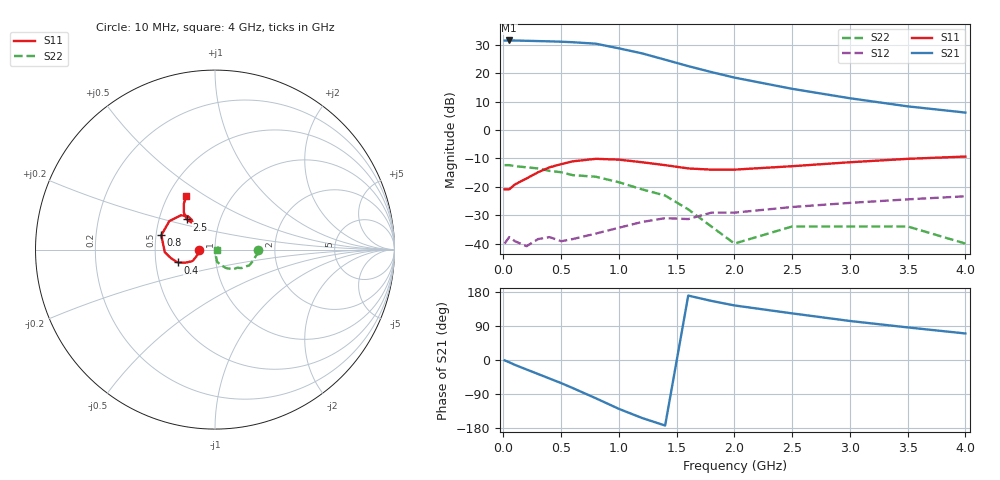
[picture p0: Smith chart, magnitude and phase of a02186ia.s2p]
!  INA-02186  S PARAMETERS
!  Id = 35 mA  LAST UPDATED 07-22-92
# ghz s ma r 50
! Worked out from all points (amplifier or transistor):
!   19 points, 10 MHz to 4 GHz, reference 50 ohm
!   highest |S21| = 31.5 dB at 50 MHz (marker M1)
!   |S21| within 3 dB of that: start of sweep to 1.025 GHz
!   unconditionally stable (mu >= 1): start of sweep to end of sweep
!   at 200 MHz: K = 1.59, MAG = 31.6 dB, |S12| = -40.9 dB
!   at 1 GHz: K = 1.16, MAG = 29.2 dB, |S12| = -34.4 dB
!   at 4 GHz: K = 3.28, MAG = 6.7 dB, |S12| = -23.3 dB
!   S11 on the Smith chart (normalised r, x): 10 MHz: 0.83, -0.01; 400 MHz: 0.65, -0.10; 800 MHz: 0.53, +0.09; 2.5 GHz: 0.69, +0.25; 4 GHz: 0.62, +0.42
0.01  0.09 -178.0  37.38 -1.0  0.01 1.0  0.24 -1.0
0.05  0.09 -172.0  37.55 -6.0  0.013 11.0  0.24 -5.0
0.1  0.11 -160.0  37.46 -13.0  0.011 8.0  0.23 -9.0
0.2  0.14 -153.0  37.04 -25.0  0.009 15.0  0.22 -17.0
0.3  0.18 -156.0  36.62 -37.0  0.012 1.0  0.21 -25.0
0.4  0.22 -161.0  36.2 -49.0  0.013 28.0  0.19 -30.0
0.5  0.25 -169.0  35.7 -61.0  0.011 42.0  0.18 -35.0
0.6  0.28 -177.0  34.94 -74.0  0.012 44.0  0.16 -39.0
0.8  0.31 165.0  32.93 -101.0  0.015 52.0  0.15 -47.0
1  0.3 148.0  27.26 -129.0  0.019 57.0  0.12 -59.0
1.2  0.27 135.0  22.26 -153.0  0.024 62.0  0.09 -70.0
1.4  0.24 129.0  17.22 -173.0  0.028 61.0  0.07 -80.0
1.6  0.21 128.0  13.27 170.0  0.027 62.0  0.04 -82.0
1.8  0.2 129.0  10.44 156.0  0.035 61.0  0.02 -83.0
2  0.2 131.0  8.34 144.0  0.035 63.0  0.01 -20.0
2.5  0.23 133.0  5.29 123.0  0.044 59.0  0.02 30.0
3  0.27 130.0  3.61 103.0  0.052 63.0  0.02 27.0
3.5  0.31 124.0  2.6 86.0  0.06 64.0  0.02 34.0
4  0.34 118.0  2.02 70.0  0.068 58.0  0.01 3.0
